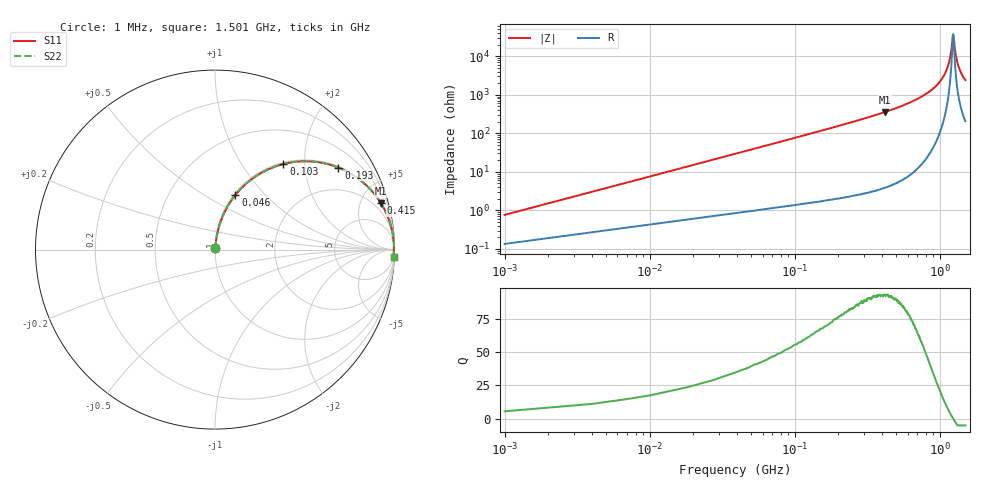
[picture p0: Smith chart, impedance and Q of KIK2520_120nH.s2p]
!version-2
!date-01.2022
!Series
# MHz S RI R 50
!Freq ReS11 ImS11 ReS21 ImS21 ReS12 ImS12 ReS22 ImS22
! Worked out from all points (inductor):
!   501 points, 1 MHz to 1.501 GHz, reference 50 ohm
!   read as one part in series: L = 120 nH near 7 MHz
!   highest Q = 92.9 at 421 MHz (marker M1), where L = 136 nH
!   self-resonance near 1.234 GHz
!   S11 on the Smith chart (normalised r, x): 1 MHz: 1.00, +0.02; 46 MHz: 1.02, +0.69; 103 MHz: 1.03, +1.56; 193 MHz: 1.04, +2.98; 415 MHz: 1.08, +7.05; 1.501 GHz: 5, -48
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1  0.00141 0.00752  0.9986 -0.00752  0.9986 -0.00752  0.00141 0.00752
10  0.00985 0.0743  0.9901 -0.0743  0.9901 -0.0743  0.00985 0.0743
16  0.0195 0.1177  0.9805 -0.1177  0.9805 -0.1177  0.0195 0.1177
28  0.049 0.1994  0.951 -0.1994  0.951 -0.1994  0.049 0.1994
46  0.1141 0.3049  0.8859 -0.3049  0.8859 -0.3049  0.1141 0.3049
103  0.3816 0.4769  0.6184 -0.4769  0.6184 -0.4769  0.3816 0.4769
193  0.6876 0.4568  0.3124 -0.4568  0.3124 -0.4568  0.6876 0.4568
253  0.7957 0.3972  0.2043 -0.3972  0.2043 -0.3972  0.7957 0.3972
415  0.9232 0.261  0.0768 -0.261  0.0768 -0.261  0.9232 0.261
421  0.9256 0.257  0.0744 -0.257  0.0744 -0.257  0.9256 0.257
502  0.9514 0.2094  0.0486 -0.2094  0.0486 -0.2094  0.9514 0.2094
751  0.9858 0.1096  0.0141 -0.1096  0.0141 -0.1096  0.9858 0.1096
1003  0.9958 0.0449  0.00421 -0.0449  0.00421 -0.0449  0.9958 0.0449
1090  0.9969 0.027  0.00308 -0.027  0.00308 -0.027  0.9969 0.027
1153  0.9973 0.0149  0.00272 -0.0149  0.00272 -0.0149  0.9973 0.0149
1192  0.9973 0.00782  0.00266 -0.00782  0.00266 -0.00782  0.9973 0.00782
1234  0.9973 0.000426  0.00272 -0.000426  0.00272 -0.000426  0.9973 0.000426
1252  0.9972 -0.00266  0.00278 0.00266  0.00278 0.00266  0.9972 -0.00266
1288  0.997 -0.00871  0.00295 0.00871  0.00295 0.00871  0.997 -0.00871
1336  0.9967 -0.0165  0.0033 0.0165  0.0033 0.0165  0.9967 -0.0165
1408  0.996 -0.0277  0.00404 0.0277  0.00404 0.0277  0.996 -0.0277
1501  0.9947 -0.0413  0.00532 0.0413  0.00532 0.0413  0.9947 -0.0413
